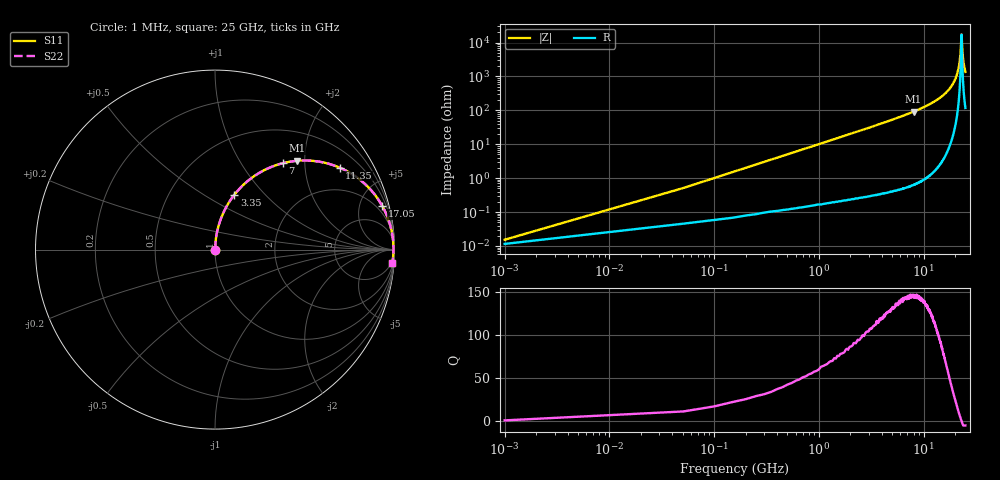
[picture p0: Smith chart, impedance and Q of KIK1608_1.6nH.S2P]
!version-2
!date-01.2022
!Series
# MHz S RI R 50
!Freq ReS11 ImS11 ReS21 ImS21 ReS12 ImS12 ReS22 ImS22
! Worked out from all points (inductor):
!   501 points, 1 MHz to 25 GHz, reference 50 ohm
!   read as one part in series: L = 1.6 nH near 101 MHz
!   highest Q = 146 at 8 GHz (marker M1), where L = 1.82 nH
!   self-resonance near 22.95 GHz
!   S11 on the Smith chart (normalised r, x): 1 MHz: 1.00, +0.00; 3.35 GHz: 1.01, +0.69; 7 GHz: 1.01, +1.55; 11.35 GHz: 1.02, +3.02; 17.05 GHz: 1.13, +7.63; 25 GHz: 3, -27
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1  0.00013 0.000101  0.9999 -0.000101  0.9999 -0.000101  0.00013 0.000101
151  0.000924 0.0152  0.9991 -0.0152  0.9991 -0.0152  0.000924 0.0152
301  0.00186 0.0302  0.9981 -0.0302  0.9981 -0.0302  0.00186 0.0302
551  0.0043 0.0551  0.9957 -0.0551  0.9957 -0.0551  0.0043 0.0551
1000  0.0117 0.0995  0.9883 -0.0995  0.9883 -0.0995  0.0117 0.0995
1550  0.0259 0.1523  0.9741 -0.1523  0.9741 -0.1523  0.0259 0.1523
3350  0.1081 0.306  0.8919 -0.306  0.8919 -0.306  0.1081 0.306
4200  0.1623 0.3647  0.8377 -0.3647  0.8377 -0.3647  0.1623 0.3647
7000  0.3766 0.4811  0.6234 -0.4811  0.6234 -0.4811  0.3766 0.4811
8000  0.4562 0.4946  0.5438 -0.4946  0.5438 -0.4946  0.4562 0.4946
8350  0.4835 0.4963  0.5165 -0.4963  0.5165 -0.4963  0.4835 0.4963
11350  0.6937 0.4571  0.3063 -0.4571  0.3063 -0.4571  0.6937 0.4571
12550  0.7619 0.4216  0.2381 -0.4216  0.2381 -0.4216  0.7619 0.4216
16700  0.9233 0.2581  0.0767 -0.2581  0.0767 -0.2581  0.9233 0.2581
17050  0.932 0.2431  0.068 -0.2431  0.068 -0.2431  0.932 0.2431
19250  0.9723 0.1489  0.0277 -0.1489  0.0277 -0.1489  0.9723 0.1489
20850  0.9879 0.0826  0.0121 -0.0826  0.0121 -0.0826  0.9879 0.0826
22150  0.9935 0.0312  0.00646 -0.0312  0.00646 -0.0312  0.9935 0.0312
22500  0.9941 0.0178  0.00589 -0.0178  0.00589 -0.0178  0.9941 0.0178
22950  0.9943 0.000822  0.0057 -0.000822  0.0057 -0.000822  0.9943 0.000822
23750  0.9933 -0.0285  0.00674 0.0285  0.00674 0.0285  0.9933 -0.0285
25000  0.9884 -0.072  0.0116 0.072  0.0116 0.072  0.9884 -0.072
